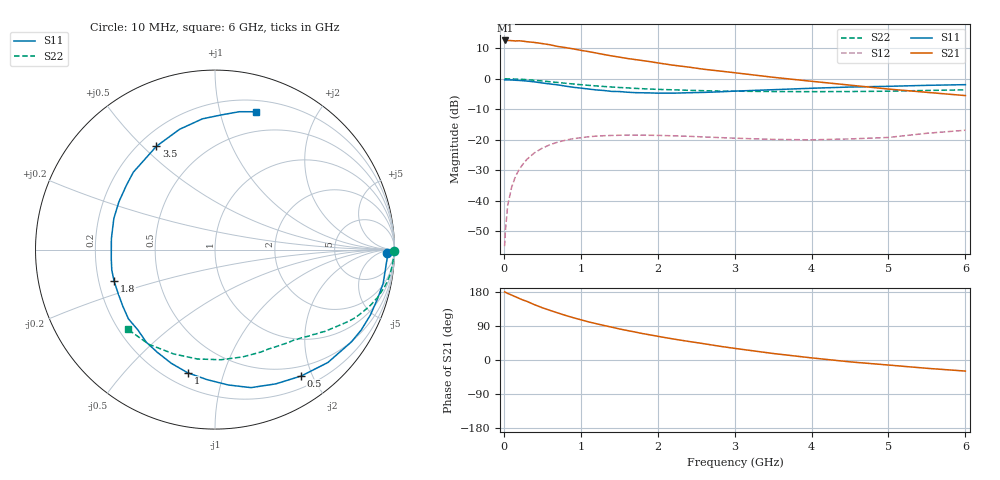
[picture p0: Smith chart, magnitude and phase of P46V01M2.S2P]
! SIEMENS Small Signal Semiconductors
! BFP182
! Si NPN RF Bipolar Junction Transistor in SOT143
! VCE = 6 V  IC = 1.2 mA
! Common Emitter S-Parameters:  March  1996
# GHz  S  MA  R  50
!  f  S11  S21  S12  S22
! GHz  MAG  ANG  MAG  ANG  MAG  ANG  MAG  ANG
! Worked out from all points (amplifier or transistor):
!   36 points, 10 MHz to 6 GHz, reference 50 ohm
!   highest |S21| = 12.6 dB at 20 MHz (marker M1)
!   |S21| within 3 dB of that: start of sweep to 951.6 MHz
!   unconditionally stable (mu >= 1): 2.547 GHz to end of sweep
!   at 250 MHz: K = 0.09, MSG = 20.1 dB, |S12| = -27.9 dB
!   at 1.4 GHz: K = 0.56, MSG = 13.0 dB, |S12| = -18.6 dB
!   at 6 GHz: K = 1.04, MAG = 4.4 dB, |S12| = -16.9 dB
!   S11 on the Smith chart (normalised r, x): 10 MHz: 40, -18; 500 MHz: 0.36, -1.84; 1 GHz: 0.28, -0.76; 1.8 GHz: 0.26, -0.14; 3.5 GHz: 0.27, +0.55; 6 GHz: 0.30, +1.29
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0.01  0.9593 -1.1  4.237 179.5  0.0018 89.6  0.9975 -0.4
0.02  0.9618 -2.2  4.247 178.9  0.0032 79.7  0.9999 -0.9
0.05  0.9564 -5.8  4.244 175.7  0.0084 91.2  0.9965 -2.1
0.1  0.9558 -11.4  4.221 171.4  0.0164 81.5  0.9924 -4.4
0.15  0.9456 -17.3  4.168 167.0  0.0249 78.9  0.9884 -6.4
0.2  0.939 -23.0  4.197 162.5  0.0327 75.7  0.9836 -8.5
0.3  0.9176 -34.1  4.051 154.7  0.0478 69.4  0.966 -12.6
0.4  0.8896 -45.0  3.933 145.8  0.0613 62.6  0.945 -16.3
0.5  0.8524 -55.7  3.773 137.9  0.0729 56.6  0.9196 -19.8
0.6  0.8213 -65.6  3.609 131.0  0.0829 51.0  0.8934 -22.9
0.8  0.7578 -84.4  3.247 117.8  0.0983 41.2  0.8452 -28.2
1  0.7033 -102.4  2.926 106.2  0.1078 33.1  0.7989 -32.6
1.1  0.6785 -111.1  2.793 100.7  0.1119 29.5  0.7804 -34.6
1.3  0.6424 -126.6  2.5 91.2  0.1165 23.4  0.7472 -38.2
1.5  0.6176 -141.4  2.266 82.1  0.1184 18.4  0.7192 -41.3
1.8  0.5891 -162.6  1.991 69.9  0.1189 12.7  0.6872 -45.7
2.2  0.5805 174.0  1.669 55.5  0.116 6.7  0.6591 -51.9
2.8  0.6098 144.1  1.343 36.5  0.1086 2.7  0.6287 -61.9
3.5  0.6619 119.5  1.058 17.2  0.1013 3.0  0.6175 -75.6
4.5  0.7319 95.5  0.786 -4.9  0.1032 10.5  0.6173 -99.2
5.5  0.7801 80.0  0.599 -21.9  0.1277 16.9  0.6433 -124.8
6  0.8006 73.6  0.53 -29.2  0.1431 15.5  0.6581 -137.5
